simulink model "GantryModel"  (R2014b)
settings: Solver=ode45  StartTime=0.0  StopTime=10.0  RelTol=1e-3
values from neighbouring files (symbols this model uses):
  C = [0 0 1 0]    [CarSuspData.m]    (also in GantryData.m)
  g = 9.8    [GantryData.m]
  l = 2    [GantryData.m]
  mc = 10    [GantryData.m]
  ml = 8    [GantryData.m]

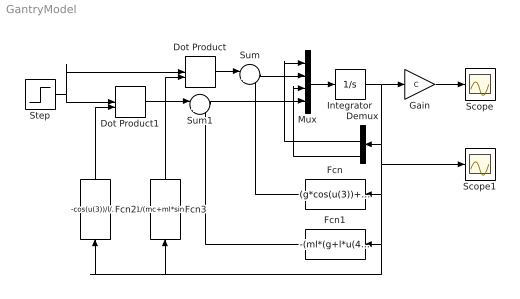
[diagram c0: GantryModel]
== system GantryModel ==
  Demux : Demux
  Dot Product : DotProduct
  Dot Product1 : DotProduct
  Fcn : Fcn  Expr=(g*cos(u(3))+l*u(4)*u(4))*ml*sin(u(3))/(mc+ml*sin(u(3))*sin(u(3)))
  Fcn1 : Fcn  Expr=-(ml*(g+l*u(4)*u(4)*cos(u(3)))+g*mc)*ml*sin(u(3))/l/(mc+ml*sin(u(3))*sin(u(3)))
  Fcn2 : Fcn  Expr=-cos(u(3))/l/(mc+ml*sin(u(3))*sin(u(3)))
  Fcn3 : Fcn  Expr=1/(mc+ml*sin(u(3))*sin(u(3)))
  Gain : Gain  Gain=C  Multiplication=Matrix(K*u) (u vector)
  Integrator : Integrator  InitialCondition=[0,0,0,0]
  Mux : Mux
  Scope : Scope
  Scope1 : Scope
  Step : Step  After=78  SampleTime=0
  Sum : Sum  Inputs=|++
  Sum1 : Sum  Inputs=|++
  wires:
  Step/1 -> Dot Product/1, Dot Product1/1
  Fcn2/1 -> Dot Product1/2
  Dot Product1/1 -> Sum1/1
  Dot Product/1 -> Sum/1
  Fcn3/1 -> Dot Product/2
  Sum/1 -> Mux/2
  Sum1/1 -> Mux/4
  Mux/1 -> Integrator/1
  Gain/1 -> Scope/1
  Fcn/1 -> Sum/2
  Fcn1/1 -> Sum1/2
  Demux/4 -> Mux/3
  Demux/2 -> Mux/1
  Integrator/1 -> Fcn2/1, Fcn3/1, Fcn1/1, Fcn/1, Scope1/1, Demux/1, Gain/1
